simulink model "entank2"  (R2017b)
settings: Solver=VariableStepAuto  StartTime=0.0  StopTime=50.0  RelTol=1e-3
libraries: simulink x1

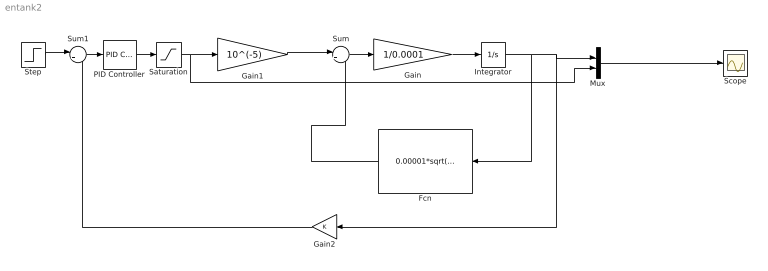
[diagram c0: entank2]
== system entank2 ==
  Fcn : Fcn  Expr=0.00001*sqrt(2*9.81*u(1))
  Gain : Gain  Gain=1/0.0001
  Gain1 : Gain  Gain=10^(-5)
  Gain2 : Gain
  Integrator : Integrator
  Mux : Mux  Inputs=2
  PID Controller : simulink/Continuous/PID Controller  Controller=PID  TimeDomain=Continuous-time  SampleTime=-1  IntegratorMethod=Forward Euler  FilterMethod=Forward Euler  Form=Parallel  UseFilter=on  ControllerParametersSource=internal  P=4  I=1  D=0  N=100  InitialConditionSource=internal  InitialConditionForIntegrator=0  InitialConditionForFilter=0  ExternalReset=none  LimitOutput=off  UpperSaturationLimit=inf  LowerSaturationLimit=-inf  LinearizeAsGain=on  AntiWindupMode=none  Kb=1  TrackingMode=off  Kt=1  PParamMin=[]  PParamMax=[]  IParamMin=[]  IParamMax=[]  DParamMin=[]  DParamMax=[]  NParamMin=[]  NParamMax=[]  KbParamMin=[]  KbParamMax=[]  KtParamMin=[]  KtParamMax=[]  POutMin=[]  POutMax=[]  IOutMin=[]  IOutMax=[]  DOutMin=[]  DOutMax=[]  NOutMin=[]  NOutMax=[]  KbOutMin=[]  KbOutMax=[]  KtOutMin=[]  KtOutMax=[]  IntegratorOutMin=[]  IntegratorOutMax=[]  FilterOutMin=[]  FilterOutMax=[]  SumOutMin=[]  SumOutMax=[]  SumI1OutMin=[]  SumI1OutMax=[]  SumI2OutMin=[]  SumI2OutMax=[]  SumI3OutMin=[]  SumI3OutMax=[]  SumDOutMin=[]  SumDOutMax=[]  SaturationOutMin=[]  SaturationOutMax=[]  IntegratorContinuousStateAttributes=''  IntegratorStateMustResolveToSignalObject=off  IntegratorRTWStateStorageClass=Auto  FilterContinuousStateAttributes=''  FilterStateMustResolveToSignalObject=off  FilterRTWStateStorageClass=Auto  DifferentiatorICPrevScaledInput=0  DifferentiatorOutMin=[]  DifferentiatorOutMax=[]  InitialConditionSetting=State (most efficient)  FilterDiffOutCoefMin=[]  FilterDiffOutCoefMax=[]  SumDenOutMin=[]  SumDenOutMax=[]  SumNumOutMin=[]  SumNumOutMax=[]  ReciprocalOutMin=[]  ReciprocalOutMax=[]  DivideOutMin=[]  DivideOutMax=[]  TunerSelectOption=Transfer Function Based (PID Tuner App)
  Saturation : Saturate  UpperLimit=5  LowerLimit=0
  Scope : Scope
  Step : Step  Time=0  SampleTime=0
  Sum : Sum  Inputs=|+-
  Sum1 : Sum  Inputs=|+-
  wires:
  PID Controller/1 -> Saturation/1
  Step/1 -> Sum1/1
  Sum1/1 -> PID Controller/1
  Gain2/1 -> Sum1/2
  Mux/1 -> Scope/1
  Saturation/1 -> Mux/2, Gain1/1
  Sum/1 -> Gain/1
  Gain/1 -> Integrator/1
  Fcn/1 -> Sum/2
  Integrator/1 -> Fcn/1, Gain2/1, Mux/1
  Gain1/1 -> Sum/1
